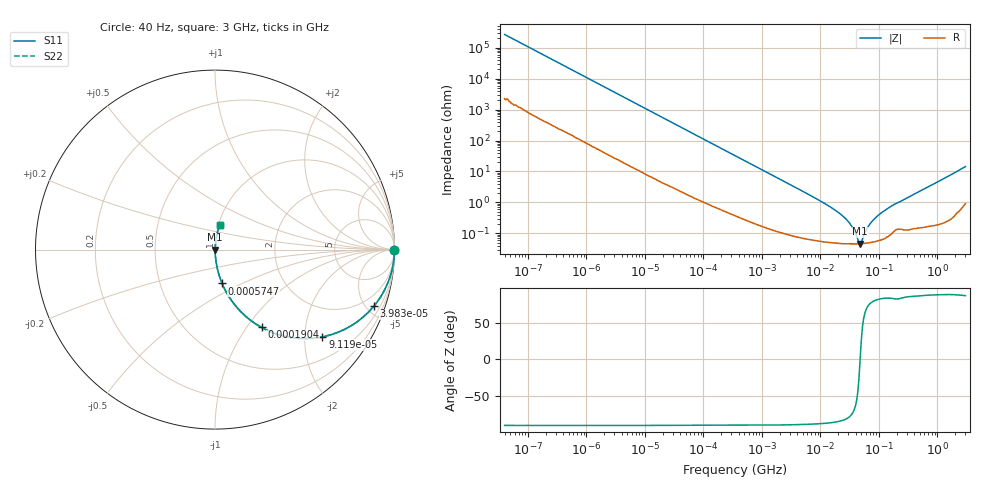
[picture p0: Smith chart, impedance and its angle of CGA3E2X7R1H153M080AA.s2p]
! S-parameter Generated by TDK Corporation
! Copyright(C) 2015 TDK Corporation.
! All Rights Reserved.
! TDK P/N: CGA3E2X7R1H153M080AA (Multilayer Ceramic Chip Capacitors)
! Property: C=15nF
! Size(LxWxT): 1.6x0.8x0.8mm, 0.063x0.031x0.031inches
! Model Type: s2p (Touchstone File Format Version 1.0)
! Frequency: DC=Yes Start=0.00004MHz Stop=3000MHz 396points Log-sweep
! Note: This model was converted from impedance.
! Model Generated on Jun. 23, 2015
! Hash(MD5):
! Port Assignments:
!  1 ---| |--- 2
! Applicable Conditions:
!  Temperature = 25 degC
!  DC Bias Voltage = 0 V
!  Small Signal Operation
! Terms and conditions regarding TDK Simulation Models
! (1)This simulation model is being provided solely for informational purposes. Please refer to the specifications of the products in terms of detailed characteristics of such products.
! (2)In no event shall TDK Corporation of any of its subsidiaries be liable for any loss or damage arising, directly or indirectly,
!  From any information contained in this simulation model, including, but not limited to loss or damages arising from any inaccuracies, omissions or errors in connection with such information.
! (3)Any and all copyrights on this simulation model are owned by TDK Corporation.
!  Duplication or redistribution of this simulation model without prior written permission from TDK Corporation is prohibited.
! (4)This simulation model is subject to any modification or change without any prior notice.
! (5)Neither TDK Corporation nor any of its subsidiaries shall make any warranty, express or implied,
!  Including but not limited to the correctness, implied warranties of merchantability and fitness for a particular purpose with respect to this simulation models.
! (6)The use of this simulation model shall be deemed to have consented to the terms and conditions hereof.
# MHz S MA R 50
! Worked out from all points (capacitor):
!   395 points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, 40 Hz to 3 GHz, reference 50 ohm
!   read as one part in series: C = 14.8 nF near 41.88 Hz
!   lowest |Z| = 46.2 mohm at 47.67 MHz (marker M1)
!   series resonance near 47.63 MHz, so ESL is about 750 pH
!   S11 on the Smith chart (normalised r, x): 40 Hz: open; 39.83 kHz: 1.05, -5.58; 91.19 kHz: 1.02, -2.45; 190.4 kHz: 1.01, -1.18; 574.7 kHz: 1.00, -0.39; 3 GHz: 1.02, +0.29
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4e-05  1 -0.0  0.0003736 89.5  0.0003736 89.5  1 -0.0
0.000834128  0.9999 -0.4  0.00765 89.1  0.00765 89.1  0.9999 -0.4
0.005256919  0.9985 -2.7  0.0477 86.8  0.0477 86.8  0.9985 -2.7
0.01739424  0.9867 -8.9  0.1551 80.6  0.1551 80.6  0.9867 -8.9
0.0398272  0.9389 -19.7  0.3366 69.9  0.3366 69.9  0.9389 -19.7
0.09119145  0.7709 -39.1  0.6301 50.4  0.6301 50.4  0.7709 -39.1
0.190438  0.5049 -59.1  0.858 30.3  0.858 30.3  0.5049 -59.1
0.3464102  0.3079 -71.4  0.9479 17.9  0.9479 17.9  0.3079 -71.4
0.5747153  0.1924 -78.2  0.9789 11.1  0.9789 11.1  0.1924 -78.2
1.656397  0.06845 -85.1  0.9965 3.9  0.9965 3.9  0.06845 -85.1
7.22376  0.0156 -86.9  0.9993 0.9  0.9993 0.9  0.0156 -86.9
15.79611  0.006555 -85.3  0.9995 0.4  0.9995 0.4  0.006555 -85.3
26.2067  0.00313 -81.4  0.9995 0.2  0.9995 0.2  0.00313 -81.4
36.16801  0.00144 -71.5  0.9995 0.1  0.9995 0.1  0.00144 -71.5
45.52626  0.0005086 -25.7  0.9995 0.0  0.9995 0.0  0.0005086 -25.7
47.67047  0.0004618 0.5  0.9995 -0.0  0.9995 -0.0  0.0004618 0.5
60.0049  0.001242 67.1  0.9995 -0.1  0.9995 -0.1  0.001242 67.1
72.13343  0.002156 76.3  0.9995 -0.1  0.9995 -0.1  0.002156 76.3
95.07391  0.003693 80.9  0.9994 -0.2  0.9994 -0.2  0.003693 80.9
150.6385  0.006956 82.6  0.9991 -0.4  0.9991 -0.4  0.006956 82.6
994.0817  0.04538 85.0  0.9971 -2.6  0.9971 -2.6  0.04538 85.0
3000  0.141 78.3  0.9811 -8.1  0.9811 -8.1  0.141 78.3
